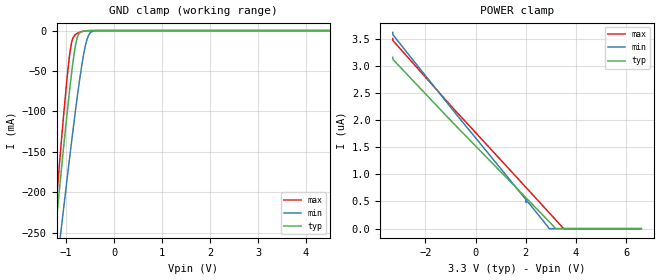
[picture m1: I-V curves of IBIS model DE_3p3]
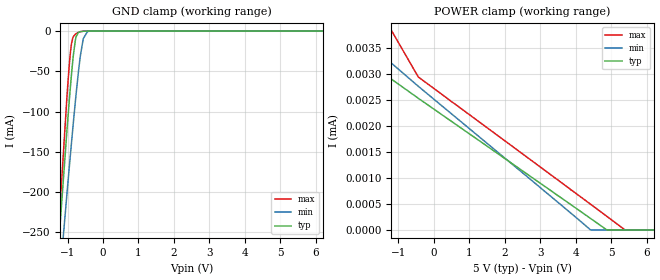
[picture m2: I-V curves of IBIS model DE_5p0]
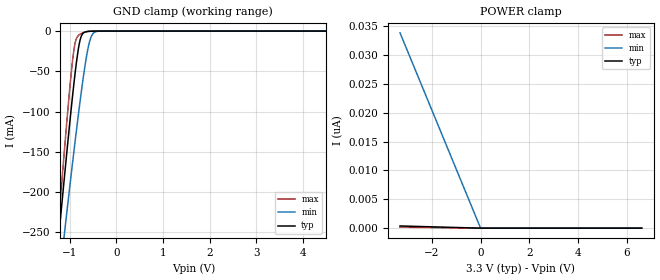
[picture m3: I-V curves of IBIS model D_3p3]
|Texas Instruments Incorporated
|THVD14x9 3.3-V to 5-V RS-485 Transceivers With Surge Protection
[IBIS Ver]   4.1
[File name]   thvd1419.ibs
[Date]   11/29/2018
[File Rev]   1.0
[Source]
| Texas Instruments Incorporated.
| Analog-eLab Design Center, HPA
| 12500 TI Blvd
| Dallas, TX -75243
[Notes]   Revision History:
| Rev 1.0: 11/29/2018
| - Initial version of the model
| - Model generated from simulations in SPECTRE
| - Warnings regarding combined Non-monotonicity of various models
|   have been reviewed and considered minor and can be ignored.
| - Model names with a trailing _3p3 contain the model for 3.3V operation.
| - Model names with a trailing _5p0 contain the model for 5.0V operation.
| - Connect 1uF capacitor at the common mode node for FAST PVT corner of
|   "diffout_5p0" model.
| - C_comp although listed in numerical order of value are
|   obtained from varying PVT conditions. For PVT conditions for
|   each specific value refer the buffer description under
|   respective [Model]. IBIS model user is responsible for using
|   appropriate C_comp to simulate for Signal Integrity.
[Disclaimer]
| This model is designed as an aid for customers of Texas Instruments.
| TI and its licensors and suppliers make no warranties, either expressed
| or implied, with respect to this  model, including the warranties of
| merchantability or fitness for a particular purpose. The model is
| provided solely on an "as is" basis. The entire risk as to its quality
| and performance is with the customer.
| This model is subject to change without notice. Texas Instruments
| Incorporated is not responsible for updating this model.
[Copyright]
(C) Copyright 2018 Texas Instruments Incorporated.All rights reserved.
|  Component THVD1419D 8-pin SOIC - D package
|  Part # THVD1419D
[Component]   THVD1419D
[Manufacturer]  TI
[Package]   |8 SOIC - D package
|   typ   min   max
R_pkg   0.05   0.04   0.06
L_pkg   1.0nH   0.8nH   1.2nH
C_pkg   0.2pF   0.16pF   0.24pF
[Pin]  signal_name  model_name   R_pin   L_pin   C_pin
1   R   R   NA   NA   NA
2   _RE   REB   NA   NA   NA
3   DE   DE   NA   NA   NA
4   D   D   NA   NA   NA
5   GND   gnd   NA   NA   NA
6   A   diffout   NA   NA   NA
7   B   diffout   NA   NA   NA
8   VCC   power   NA   NA   NA
[Diff_pin]   inv_pin   vdiff   tdelay_typ   tdelay_min   tdelay_max
6   7   0.1   NA   NA   NA
|   Model Selectors
[Model Selector] DE
DE_3p3   3.3V   digital Input
DE_5p0   5.0V   digital Input
[Model Selector] D
D_3p3   3.3V   digital Input
D_5p0   5.0V   digital Input
[Model Selector] REB
REB_3p3   3.3V   digital Input
REB_5p0   5.0V   digital Input
[Model Selector] R
R_3p3   3.3V   digital Output
R_5p0   5.0V   digital Output
[Model Selector] diffout
diffout_3p3   3.3V   digital I/O
diffout_5p0   5.0V   digital I/O
| Models and submodels in the file (10): DE_3p3 (Input), DE_5p0 (Input), D_3p3 (Input), D_5p0 (Input), REB_3p3 (Input), REB_5p0 (Input), R_3p3 (3-state), R_5p0 (3-state), diffout_3p3 (I/O), diffout_5p0 (I/O)
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|   DE_3p3 Model
[Model]   DE_3p3
Model_type   Input
Vinl = 0.8
Vinh = 2
|   typ   min   max
C_comp   2.408pF   2.353pF   2.498pF
| Where Nom  PVT is Nominal Process, 3.3V, 25C
|   Fast PVT is Strong Process,  3.6V, -40C
|   Slow PVT is Weak Process,   3.0V, 150C
[Voltage Range]   3.3   3   3.6
|Junction Temperature
[Temperature Range]   25   150   -40
[Power Clamp Reference]   3.3   3   3.6
[GND Clamp Reference]   0   0   0
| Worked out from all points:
|   GND clamp passes 1 mA (typ) near -0.66 V on its own axis
[GND Clamp]
|   Voltage   I(typ)   I(min)   I(max)
-3.3V     -1.586A    -1.428A    -1.816A
-1.379V   -345mA     -389.7mA   -341.2mA
-1.221V   -246.3mA   -306.7mA   -224.2mA
-1.112V   -179.9mA   -250.5mA   -146.1mA
-993.3mV  -110.1mA   -190.2mA   -66.77mA
-914.1mV  -66.68mA   -151mA     -24.54mA
-874.5mV  -46.87mA   -131.8mA   -12.12mA
-815.1mV  -21.83mA   -103.7mA   -5.387mA
-726mV    -3.461mA   -64.12mA   -2.317mA
-567.6mV  -215.5uA   -11.52mA   -217.3uA
-399.3mV  -8.946uA   -248.4uA   -5.336uA
6.6V      0A         0A         0A
[POWER Clamp]
|   Voltage   I(typ)   I(min)   I(max)
-3.3V     3.154uA    3.612uA    3.5uA
-3.29V    3.114uA    3.569uA    3.462uA
-953.7mV  1.974uA    2.213uA    2.247uA
1.987V    578.4nA    545.9nA    769.7nA
2.006V    568.9nA    532.5nA    759.7nA
2.016V    564.2nA    481nA      754.7nA
2.026V    559.5nA    523.5nA    749.7nA
2.927V    129.8nA    3.794nA    295.2nA
3.194V    1.103nA    0A         159.8nA
3.521V    0A         0A         0A
6.6V      0A         0A         0A
|   DE_5p0 Model
[Model]   DE_5p0
Model_type   Input
Vinl = 0.8
Vinh = 2
|   typ   min   max
C_comp   2.237pF   2.186pF   2.332pF
| Where Nom  PVT is Nominal Process, 5.0V, 25C
|   Fast PVT is Strong Process,  5.5V, -40C
|   Slow PVT is Weak Process,   4.5V, 150C
[Voltage Range]   5   4.5   5.5
|Junction Temperature
[Temperature Range]   25   150   -40
[Power Clamp Reference]   5   4.5   5.5
[GND Clamp Reference]   0   0   0
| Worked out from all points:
|   GND clamp passes 1 mA (typ) near -0.66 V on its own axis
[GND Clamp]
|   Voltage   I(typ)   I(min)   I(max)
-3.4V     -1.651A    -1.483A    -1.895A
-1.252V   -265.7mA   -323.1mA   -247.1mA
-1.241V   -258.4mA   -316.9mA   -238.5mA
-1.016V   -123.3mA   -201.8mA   -81.33mA
-922mV    -70.82mA   -154.8mA   -27.91mA
-851.2mV  -36.2mA    -120.7mA   -8.298mA
-780.4mV  -11.53mA   -87.86mA   -3.903mA
-697.8mV  -1.934mA   -52.54mA   -1.689mA
-638.8mV  -695.1uA   -30.77mA   -754.3uA
-556.2mV  -177.1uA   -9.401mA   -174.2uA
-391mV    -7.477uA   -202.4uA   -4.298uA
8.4V      0A         0A         0A
[POWER Clamp]
|   Voltage   I(typ)   I(min)   I(max)
-3.4V     5.634uA    4.548uA    28.82mA
-3.093V   3.816uA    4.315uA    3.708mA
-2.904V   3.723uA    4.2uA      5.842uA
-438.2mV  2.527uA    2.757uA    2.935uA
4.412V    224.3nA    3.738nA    497.4nA
4.872V    2.638nA    0A         264.5nA
5.403V    0A         0A         0A
8.4V      0A         0A         0A
|   D_3p3 Model
[Model]   D_3p3
Model_type   Input
Vinl = 0.8
Vinh = 2
|   typ   min   max
C_comp   2.408pF   2.353pF   2.498pF
| Where Nom  PVT is Nominal Process, 3.3V, 25C
|   Fast PVT is Strong Process,  3.6V, -40C
|   Slow PVT is Weak Process,   3.0V, 150C
[Voltage Range]   3.3   3   3.6
|Junction Temperature
[Temperature Range]   25   150   -40
[Power Clamp Reference]   3.3   3   3.6
[GND Clamp Reference]   0   0   0
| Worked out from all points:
|   GND clamp passes 1 mA (typ) near -0.66 V on its own axis
[GND Clamp]
|   Voltage   I(typ)   I(min)   I(max)
-3.3V     -1.586A    -1.428A    -1.816A
-1.379V   -345mA     -389.7mA   -341.2mA
-1.221V   -246.3mA   -306.7mA   -224.2mA
-1.112V   -179.9mA   -250.5mA   -146.1mA
-993.3mV  -110.1mA   -190.2mA   -66.77mA
-914.1mV  -66.68mA   -151mA     -24.54mA
-874.5mV  -46.87mA   -131.8mA   -12.12mA
-815.1mV  -21.83mA   -103.7mA   -5.388mA
-726mV    -3.462mA   -64.12mA   -2.318mA
-567.6mV  -216.4uA   -11.52mA   -218.3uA
-399.3mV  -10.34uA   -250.2uA   -7uA
6.6V      0A         0A         0A
[POWER Clamp]
|   Voltage   I(typ)   I(min)   I(max)
-3.3V     380.5pA    33.86nA    171pA
0V        0A         0A         0A
6.6V      0A         0A         0A
